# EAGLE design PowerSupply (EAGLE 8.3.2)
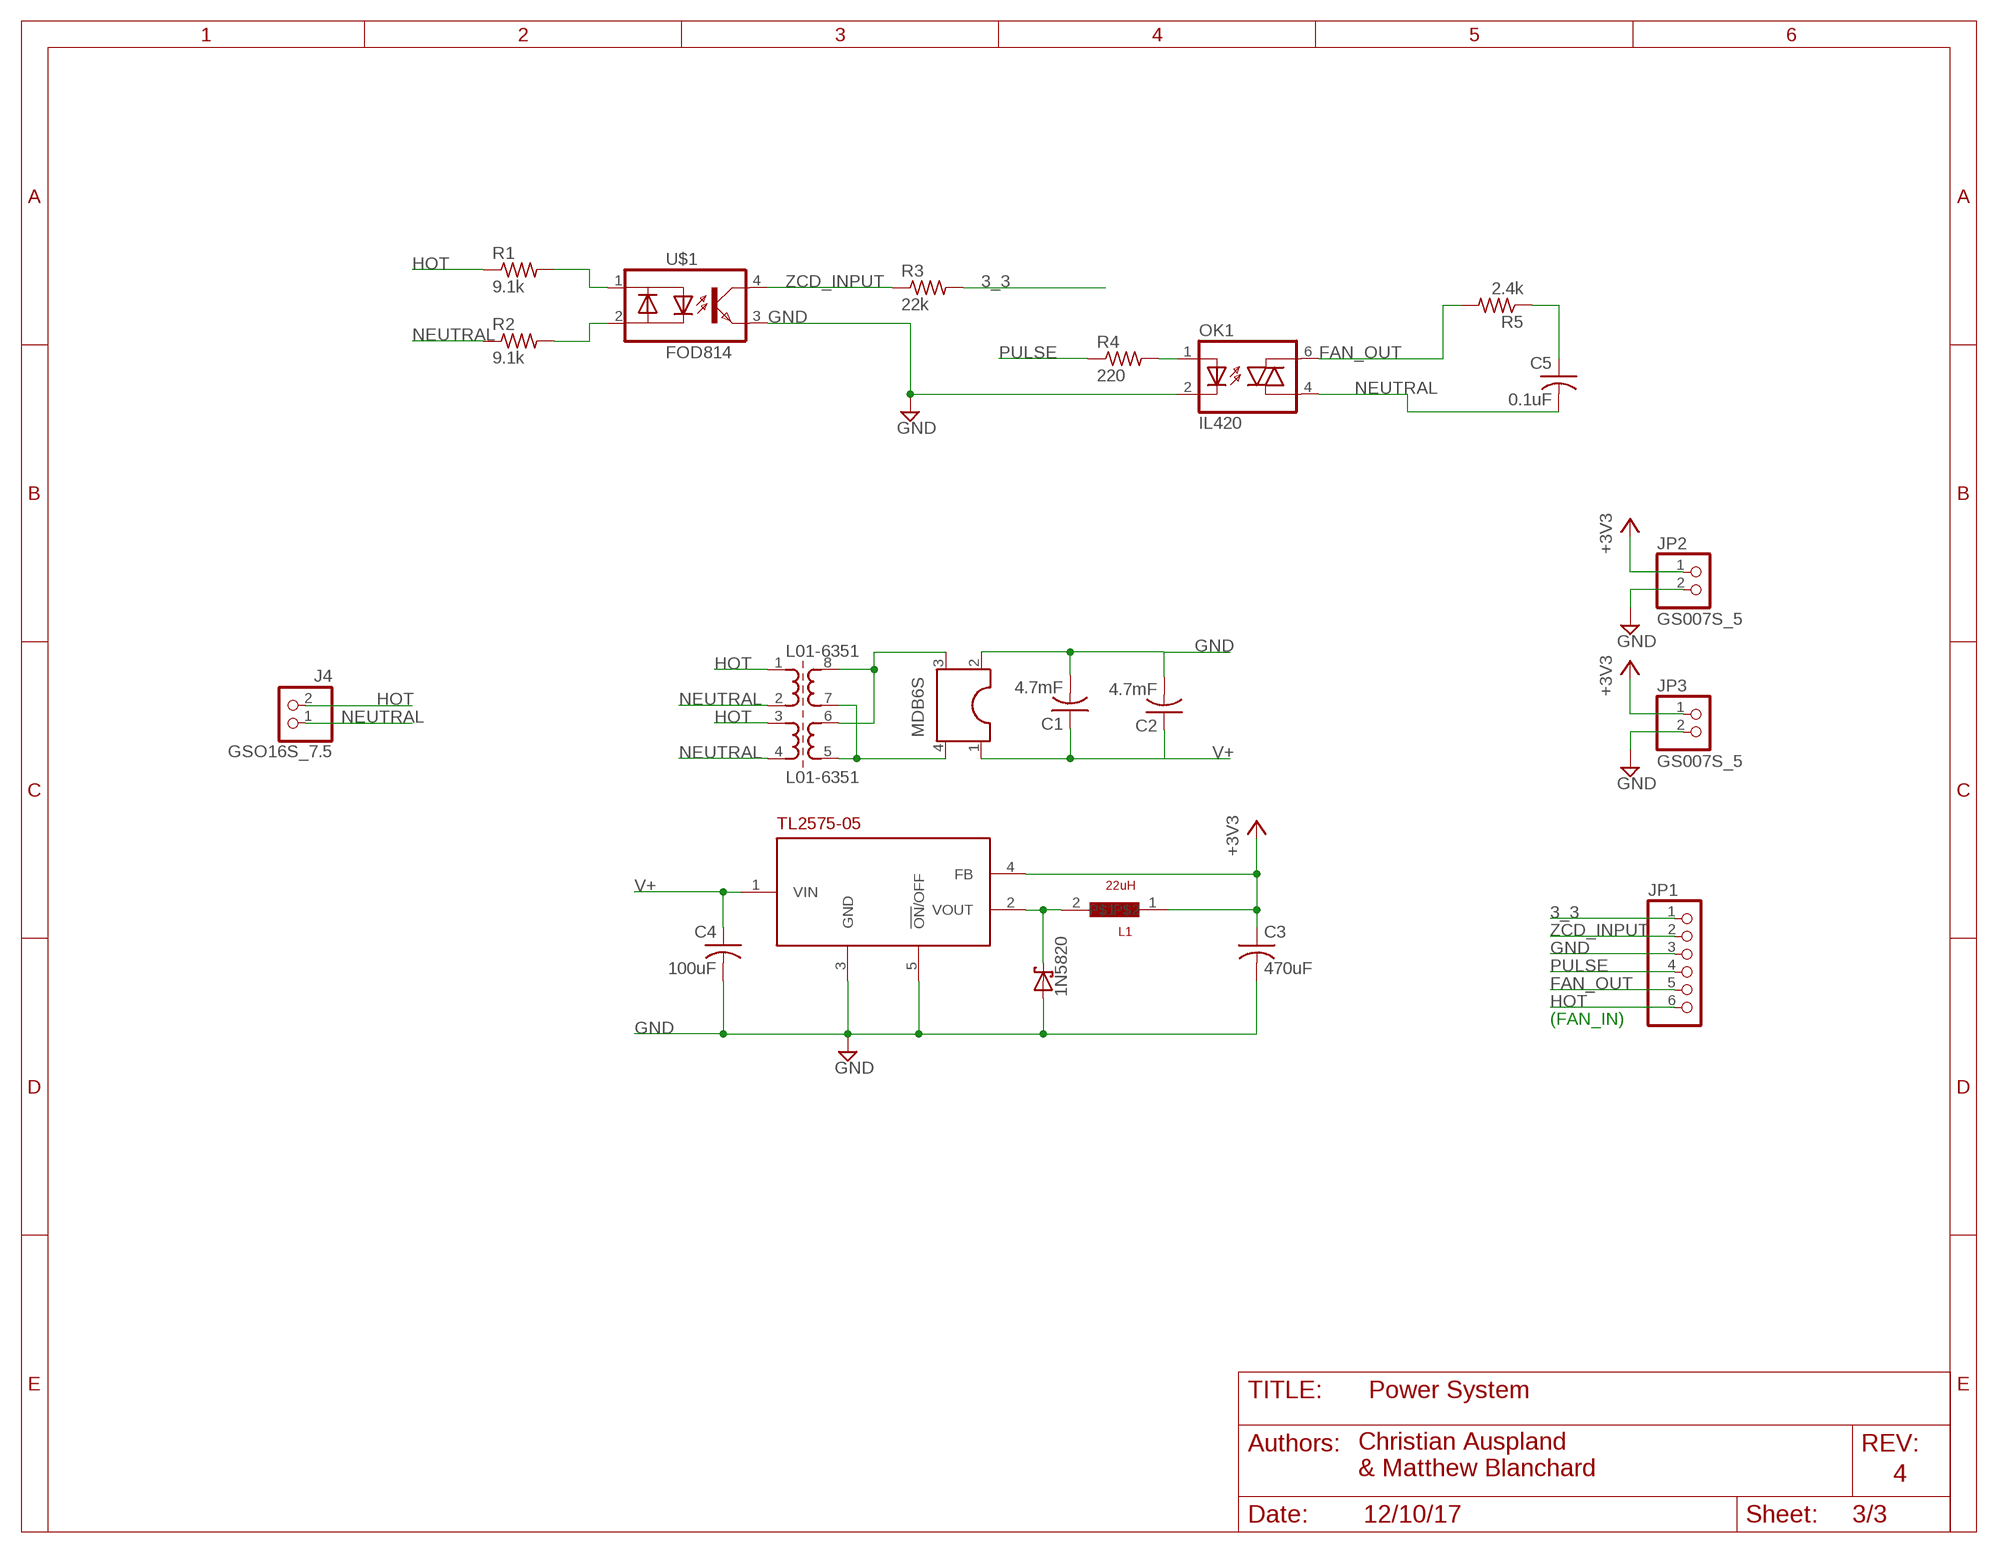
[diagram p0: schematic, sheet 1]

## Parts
1N5820  1N5820  [1N5820]
C1  4.7mF  478CKE016M  [478CKE016M]
C2  4.7mF  478CKE016M  [478CKE016M]
C3  470uF  ESW477M050AL3AA  [ESW477M050AL3AA]
C4  100uF  CAP  [MYCAP]
C5  0.1uF  CAP  [MYCAP]
GSO16S_7.5  J4  GSO16S_7.5  [GSO16S_7.5]
JP1  PINHD-1X6  [1X06]
JP2  GS007S_5  [GS007S_5]
JP3  GS007S_5  [GS007S_5]
L1  22uH  2100HT-220-RC  [2100HT-220-RC]
L01-6351  L01-6351  [L01-6351]
MDB6S  MDB6S  [MDB6S]
OK1  IL420  [DIL06]
R1  9.1k  2WRES  [2WRES]
R2  9.1k  2WRES  [2WRES]
R3  22k  R10K  [R10K]
R4  220  R10K  [R10K]
R5  2.4k  R10K  [R10K]
TL2575-05  TL2575-05  [TL2575]
U$1  FOD814  [FOD814]

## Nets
3_3: JP1.1 R3.2
+3V3: C3.P JP2.1 JP3.1 L1.1 TL2575-05.4(FB)
FAN_OUT: JP1.5 OK1.6(A2) R5.2
GND: 1N5820.A C1.2 C2.2 C3.M C4.M JP1.3 JP2.2 JP3.2 MDB6S.2 OK1.2(C) TL2575-05.3(GND) TL2575-05.5(!ON!/OFF) U$1.3
HOT: GSO16S_7.5.2 JP1.6 L01-6351.1 L01-6351.3 R1.1
N$1: L01-6351.5 L01-6351.7 MDB6S.4
N$2: L01-6351.6 L01-6351.8 MDB6S.3
N$3: R2.2 U$1.2
N$4: R1.2 U$1.1
N$5: C5.P R5.1
N$6: OK1.1(A) R4.2
N$19: 1N5820.C L1.2 TL2575-05.2(VOUT)
NEUTRAL: C5.M GSO16S_7.5.1 L01-6351.2 L01-6351.4 OK1.4(A1) R2.1
PULSE: JP1.4 R4.1
V+: C1.1 C2.1 C4.P MDB6S.1 TL2575-05.1(VIN)
ZCD_INPUT: JP1.2 R3.1 U$1.4

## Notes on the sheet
- (FAN_IN)
- Power System
- Christian Auspland
  & Matthew Blanchard
- 4
- 12/10/17 | 3/3

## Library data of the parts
1N5820 = MyLibrary:1N5820
C1 C2 = MyLibrary:478CKE016M
C3 = MyLibrary:ESW477M050AL3AA
C4 C5 = MyLibrary:CAP
GSO16S_7.5 = MyLibrary:GSO16S_7.5
JP1 = adafruit:PINHD-1X6: PIN HEADER
JP2 JP3 = MyLibrary:GS007S_5
L1 = MyLibrary:2100HT-220-RC
L01-6351 = MyLibrary:L01-6351
MDB6S = MyLibrary:MDB6S
OK1 = optocoupler:IL420: SIEMENS OPTO COUPLER; MF: VISHAY/TELEFUNKEN; MPN: IL420; OC_FARNELL: 1469561; OC_NEWARK: 58K1719
R1 R2 = MyLibrary:2WRES
R3-R5 = MyLibrary:R10K
TL2575-05 = MyLibrary:TL2575-05: TL2574 1-A SIMPLE STEP-DOWN SWITCHING VOLTAGE REGULATORS Datasheet: http://www.ti.com/lit/ds/symlink/tl2575-05.pdf
U$1 = MyLibrary:FOD814

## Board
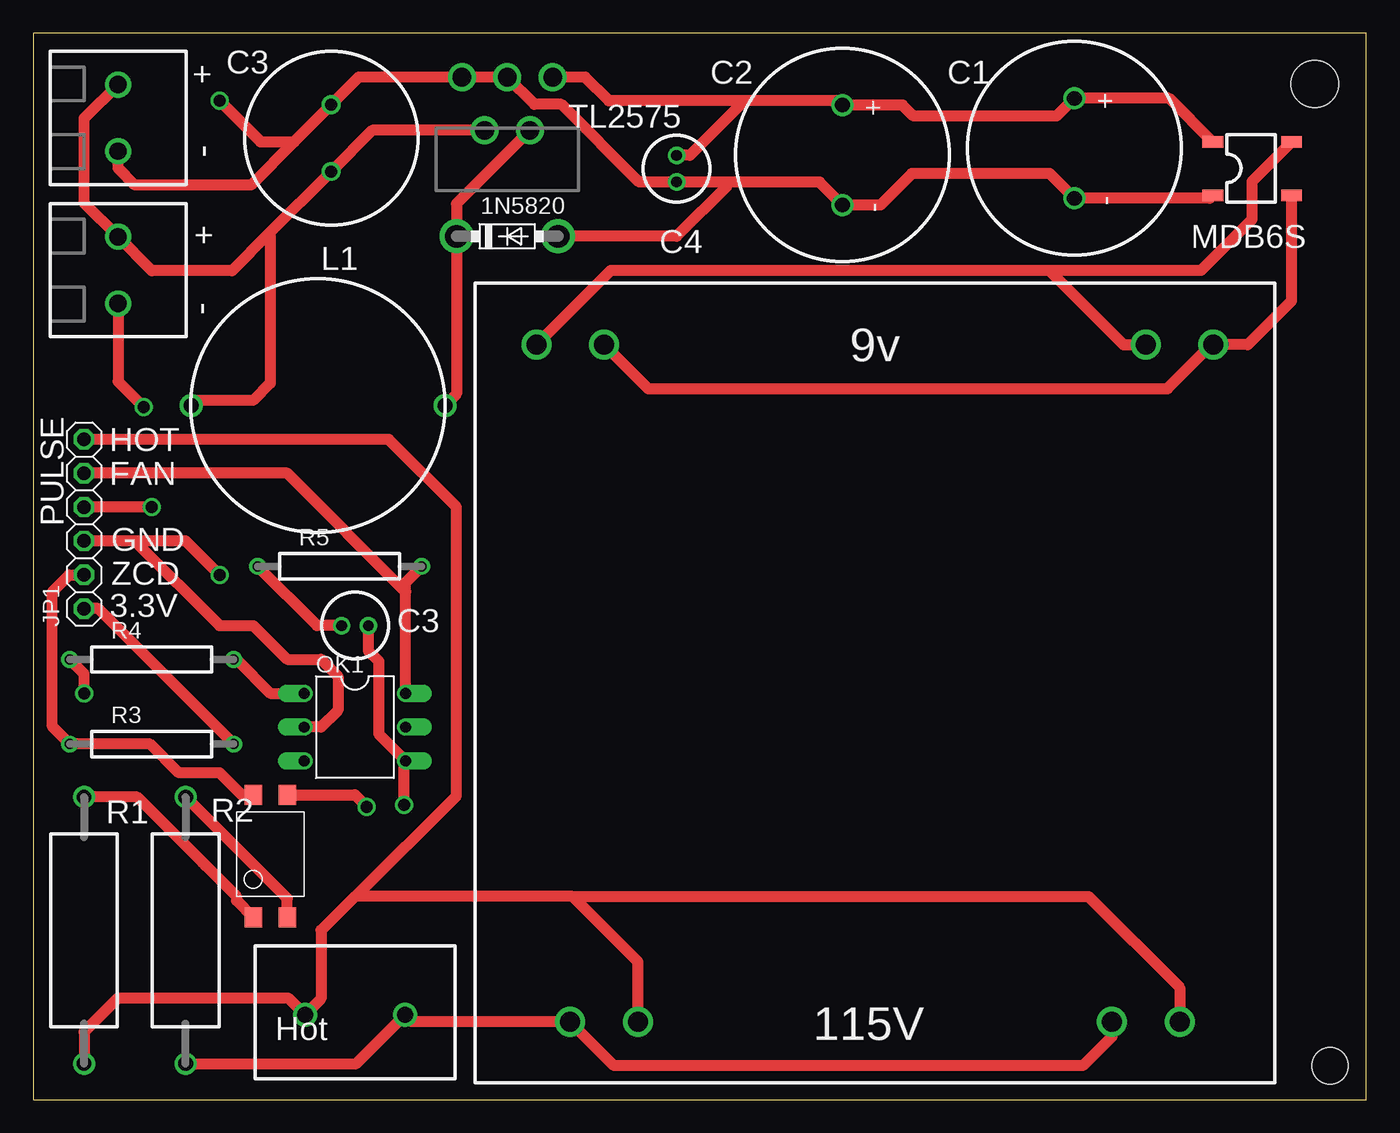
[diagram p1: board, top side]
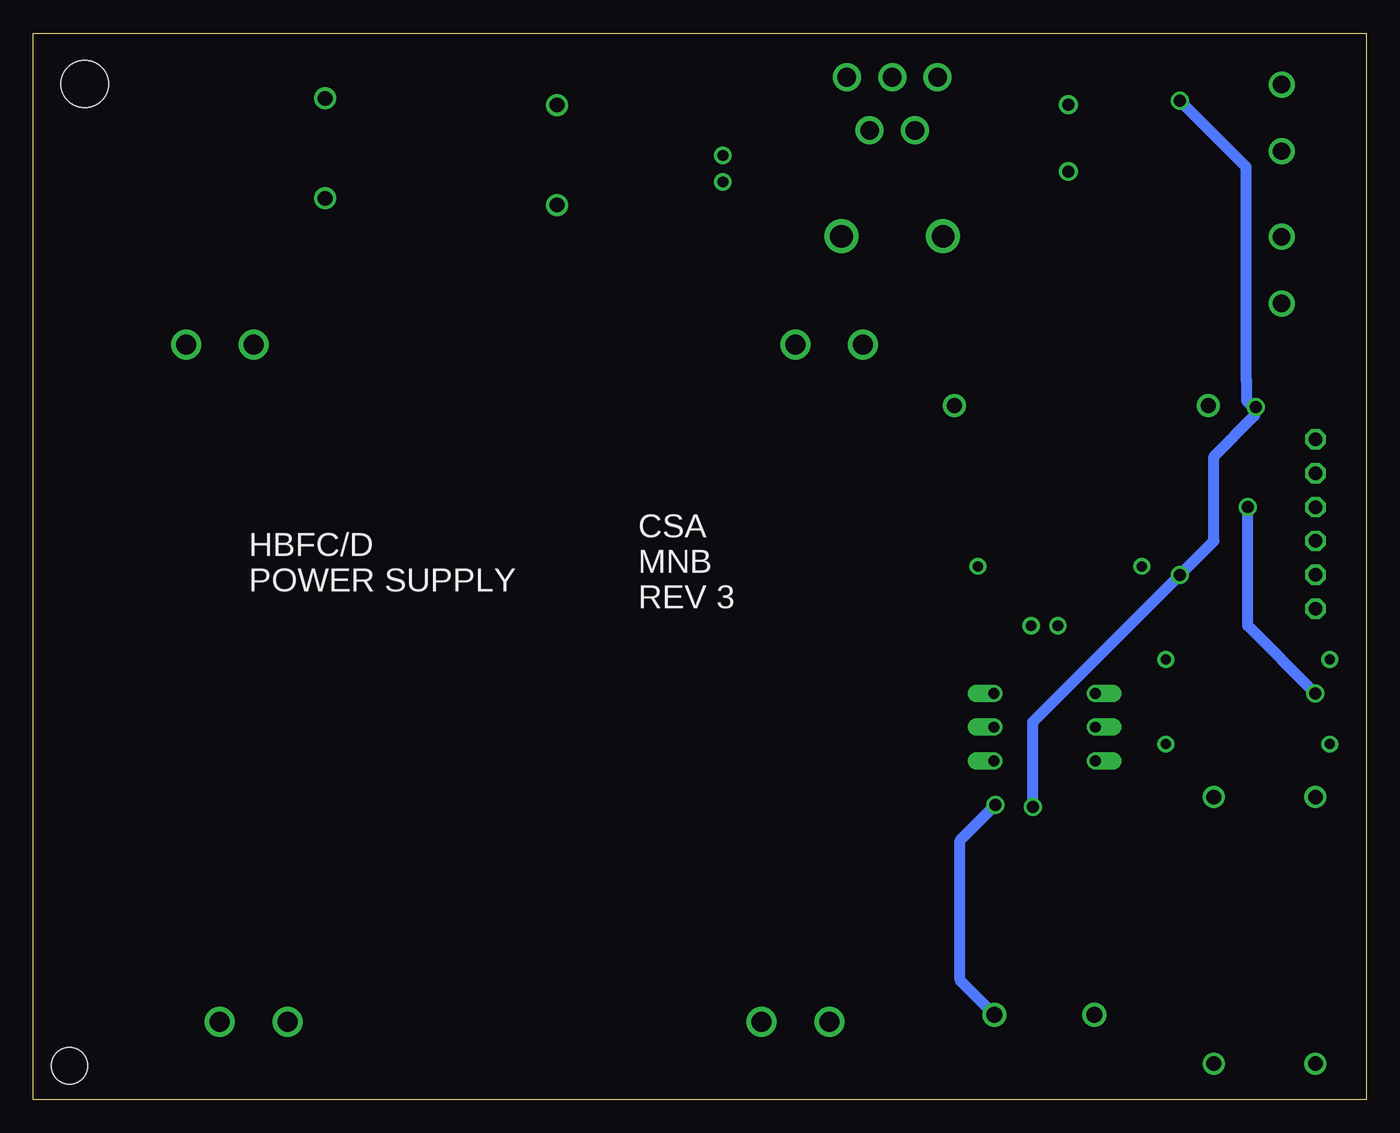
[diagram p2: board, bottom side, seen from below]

Size 100 x 80 mm. Coordinates in mm from the lower left corner, seen from the top.
Outline: 0,0 100,0 100,80 0,80 0,0
Copper layers (1*16): Top 0.035mm / dielectric 1.5mm / Bottom 0.035mm
Design rules "default *": minimum track width 10mil, minimum drill 15mil, track to track 10mil, track to pad 10mil, pad to pad 10mil, via to via 10mil, smd to smd 6mil, copper to edge 15mil, drill to drill 10mil, minimum pad ring 10mil, minimum via ring 8mil, stop-mask expansion 4mil, vias tented up to drill 0mil, thermal gap 10mil
Holes 3.56 mm at 96.14,76.2
Holes 2.73 mm at 97.28,2.54

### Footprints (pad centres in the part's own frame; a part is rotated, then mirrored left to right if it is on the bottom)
1N5820 = drill 1.7 pad 2.5: A 7.62,2.54; C 0,2.54
478CKE016M = drill 1.1: 1 -3.75,0; 2 3.75,0
ESW477M050AL3AA = drill 0.9: M 2.5,0; P -2.5,0
MYCAP = drill 0.8: M 1,0; P -1,0
GSO16S_7.5 = drill 1.2: 1 -3.75,0; 2 3.75,0
1X06 = drill 1.016 octagon: 1 -6.35,0; 2 -3.81,0; 3 -1.27,0; 4 1.27,0; 5 3.81,0; 6 6.35,0
GS007S_5 = drill 1.3: 1 -2.5,0; 2 2.5,0
2100HT-220-RC = drill 1.143: 1 -9.525,0; 2 9.525,0
L01-6351 = drill 1.5: 1 -22.86,25.4; 2 -17.78,25.4; 3 17.78,25.4; 4 22.86,25.4; 5 25.4,-25.4; 6 20.32,-25.4; 7 -20.32,-25.4; 8 -25.4,-25.4
MDB6S = smd 0.85 x 1.55: 1 -2,-2.95; 2 2,-2.95; 3 2,2.95; 4 -2,2.95
DIL06 = drill 0.813 offset: 1 -2.54,-3.81; 2 0,-3.81; 3 2.54,-3.81; 4 2.54,3.81; 5 0,3.81; 6 -2.54,3.81
2WRES = drill 1.1: 1 -10,0; 2 10,0
R10K = drill 0.75: 1 -6.15,0; 2 6.15,0
TL2575 = drill 1.397: 1 -3.404,-5.588; 2 -1.702,-1.6; 3 0,-5.588; 4 1.702,-1.6; 5 3.404,-5.588
FOD814 = smd 1.3 x 1.5: 1 2.54,9.2; 2 0,9.2; 3 0,0; 4 2.54,0

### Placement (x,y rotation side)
1N5820  31.75,62.23 0 top
C1  60.71,70.87 270 top
C2  78.11,71.37 270 top
C3  22.35,72.14 90 top
C4  48.26,69.85 270 top
C5  24.13,35.56 0 top
GSO16S_7.5  24.13,6.35 180 top
JP1  3.81,43.18 90 top
JP2  6.35,62.23 270 top
JP3  6.35,73.66 270 top
L1  21.36,52.07 0 top
L01-6351  63.14,31.24 180 top
MDB6S  91.44,69.85 270 top
OK1  24.13,27.94 270 top
R1  3.81,12.7 90 top
R2  11.43,12.7 90 top
R3  8.89,26.67 0 top
R4  8.89,33.02 0 top
R5  22.99,40.01 0 top
TL2575-05  35.56,71.12 180 top
U$1  19.05,22.86 180 top

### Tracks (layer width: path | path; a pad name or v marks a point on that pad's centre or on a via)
3_3
  Top 0.813: R3.2 4.88,36.83 JP1.1
+3V3
  Top 0.813: TL2575-05.4 25.44,72.72 C3.P 17.63,64.92 | 17.63,64.92 14.91,62.19 8.89,62.19 JP2.1 3.81,67.27 3.81,73.62 JP3.1 | 17.63,64.92 17.78,64.77 17.78,53.75 16.48,52.45 12.22,52.45 L1.1
FAN_OUT
  Top 0.813: JP1.5 19.05,46.99 27.94,38.1 | OK1.6 27.94,38.1 | 27.94,38.1 27.94,38.81 R5.2
GND  (via drill 0.9)
  Top 0.813: 52.07,68.85 58.15,68.85 58.17,68.83 58.99,68.83 C1.2 63.56,67.12 65.91,69.47 76.26,69.47 C2.2 88.26,67.62 MDB6S.2 | 52.07,68.85 C4.M 45.45,68.85 39.62,74.68 37.59,74.68 TL2575-05.3 TL2575-05.5 24.42,76.71 C3.M 19.58,71.86 | 52.07,68.85 52.07,68.58 48.26,64.77 1N5820.A | 7.62,41.91 13.97,35.56 16.51,35.56 19.05,33.02 21.59,33.02 22.86,31.75 22.86,29.21 21.59,27.94 OK1.2 | 7.62,41.91 JP1.3 | v13.97,39.37 11.43,41.91 7.62,41.91 | 19.58,71.86 16.34,68.62 7.62,68.62 6.35,69.89 JP3.2 | 19.58,71.86 17.04,71.86 v13.97,74.93 | v8.28,51.94 6.35,53.87 JP2.2 | U$1.3 24.13,22.86 v25.02,21.97
  Bottom 0.813: 8.38,51.84 8.38,51.31 11.43,48.26 11.43,41.91 v13.97,39.37 25.02,28.32 v25.02,21.97 | 8.38,51.84 v8.28,51.94 | 8.38,51.84 8.99,52.45 8.99,53.95 9.02,53.98 9.02,69.98 v13.97,74.93
HOT
  Top 0.813: R1.1 3.81,5.08 6.35,7.62 19.11,7.62 GSO16S_7.5.2 21.59,7.56 21.59,12.7 24.13,15.24 24.19,15.24 | 24.19,15.24 31.75,22.8 31.75,44.45 26.67,49.53 JP1.6 | L01-6351.1 86,8.41 79.17,15.24 40.46,15.24 | 40.46,15.24 24.19,15.24 | L01-6351.3 45.36,10.34 40.46,15.24
N$1
  Top 0.813: 76.2,62.23 43.33,62.23 L01-6351.5 | 76.2,62.23 81.79,56.64 L01-6351.7 | 76.2,62.23 87.63,62.23 91.44,66.04 91.44,68.9 MDB6S.4
N$2
  Top 0.813: L01-6351.6 46.13,53.34 85.09,53.34 88.39,56.64 L01-6351.8 91.11,56.64 94.39,59.92 MDB6S.3
N$3
  Top 0.813: U$1.2 19.05,15.08 R2.2
N$4
  Top 0.813: R1.2 7.78,22.7 12.7,17.78 | 13.01,17.47 12.7,17.78 | 12.7,17.78 15.24,15.24 15.24,14.93 U$1.1
N$5
  Top 0.813: C5.P 21.28,35.56 R5.1
N$6
  Top 0.813: R4.2 15.24,33.02 17.78,30.48 OK1.1
N$19
  Top 0.813: TL2575-05.2 31.75,67.21 1N5820.C 31.75,52.93 L1.2
NEUTRAL  (via drill 0.9)
  Top 0.813: L01-6351.2 80.92,4.72 78.74,2.54 43.59,2.54 L01-6351.4 28.39,5.84 GSO16S_7.5.1 24.23,2.7 R2.1 | C5.M 25.13,33.67 25.91,32.89 25.91,27.43 OK1.4 27.81,25.27 v27.81,22.1
  Bottom 0.813: GSO16S_7.5.1 30.48,8.95 30.48,19.43 v27.81,22.1
PULSE  (via drill 0.9)
  Top 0.813: v3.81,30.48 3.81,31.95 R4.1 | v8.89,44.45 JP1.4
  Bottom 0.813: v3.81,30.48 8.89,35.56 v8.89,44.45
V+
  Top 0.813: 53.34,74.93 60.39,74.93 C1.1 65.21,74.62 66.04,73.79 76.77,73.79 C2.1 85.22,75.12 MDB6S.1 | 53.34,74.93 49.26,70.85 C4.P | 53.34,74.93 43.18,74.93 41.4,76.71 TL2575-05.1
ZCD_INPUT
  Top 0.813: JP1.2 2.69,39.37 1.42,38.1 1.42,27.99 R3.1 8.76,26.67 10.92,24.51 13.97,24.51 15.62,22.86 U$1.4

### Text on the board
tPlace: C3 | + | C2 | C1 | TL2575 | - | + | C4 | MDB6S | L1 | - | HOT | FAN | PULSE | GND | ZCD | C3 | 3.3V | R1 | R2 | Hot
bPlace: HBFC/D / POWER SUPPLY | CSA / MNB / REV 3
